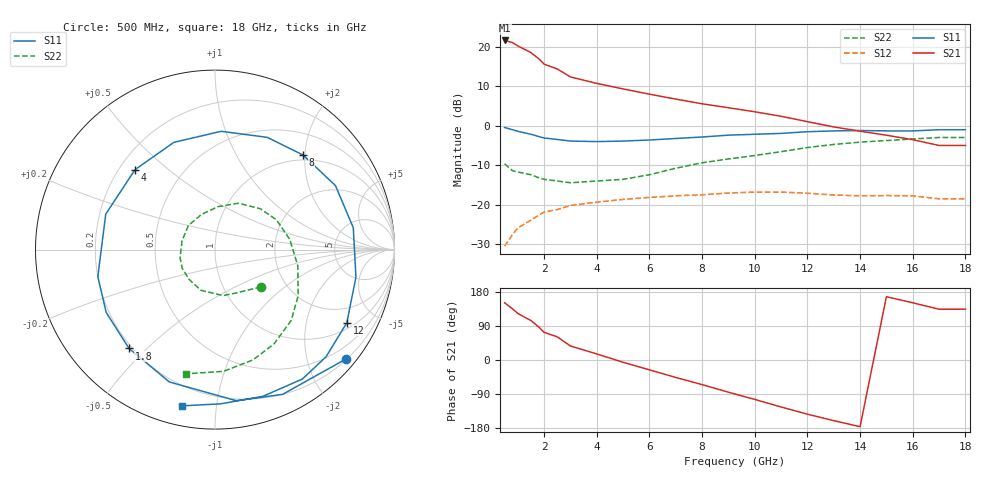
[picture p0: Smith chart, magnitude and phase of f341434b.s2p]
!ATF-34143
!S-PARAMETERS at Vds=4V  Id=40mA.  LAST UPDATED 01-29-99
# ghz s ma r 50
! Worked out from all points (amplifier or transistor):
!   23 points, 500 MHz to 18 GHz, reference 50 ohm
!   highest |S21| = 21.6 dB at 500 MHz (marker M1)
!   |S21| within 3 dB of that: start of sweep to 1.478 GHz
!   unconditionally stable (mu >= 1): 4.499 GHz to end of sweep
!   at 1.5 GHz: K = 0.42, MSG = 21.2 dB, |S12| = -23.9 dB
!   at 7 GHz: K = 1.12, MAG = 10.1 dB, |S12| = -17.7 dB
!   at 18 GHz: K = 1.33, MAG = 3.3 dB, |S12| = -18.5 dB
!   lowest NFmin = 0.10 dB at 500 MHz
!   S11 on the Smith chart (normalised r, x): 500 MHz: 0.22, -2.73; 1.8 GHz: 0.19, -0.44; 4 GHz: 0.26, +0.39; 8 GHz: 0.90, +1.96; 12 GHz: 1.25, -3.45; 18 GHz: 0.10, -0.81
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0.5  0.95 -40.0  11.97 151.0  0.03 68.0  0.33 -39.0
0.8  0.89 -65.0  11.25 135.0  0.042 56.0  0.27 -63.0
1  0.85 -82.0  10.22 123.0  0.051 48.0  0.26 -80.0
1.5  0.78 -109.0  8.405 104.0  0.064 36.0  0.24 -109.0
1.8  0.73 -131.0  7.024 87.0  0.074 27.0  0.22 -131.0
2  0.7 -150.0  6.002 73.0  0.081 19.0  0.21 -150.0
2.5  0.67 -167.0  5.223 61.0  0.087 12.0  0.2 -167.0
3  0.64 162.0  4.141 37.0  0.098 -1.0  0.19 165.0
4  0.63 135.0  3.428 16.0  0.108 -13.0  0.2 138.0
5  0.64 111.0  2.923 -6.0  0.117 -27.0  0.21 111.0
6  0.66 87.0  2.506 -26.0  0.124 -41.0  0.24 86.0
7  0.69 65.0  2.173 -46.0  0.13 -54.0  0.29 63.0
8  0.72 47.0  1.894 -65.0  0.134 -68.0  0.34 42.0
9  0.76 28.0  1.689 -85.0  0.141 -82.0  0.38 26.0
10  0.78 9.0  1.501 -104.0  0.145 -97.0  0.42 8.0
11  0.8 -11.0  1.317 -124.0  0.145 -113.0  0.47 -11.0
12  0.84 -29.0  1.125 -143.0  0.14 -128.0  0.53 -29.0
13  0.86 -44.0  0.966 -160.0  0.133 -141.0  0.58 -43.0
15  0.86 -72.0  0.759 167.0  0.131 -165.0  0.65 -71.0
16  0.86 -88.0  0.666 151.0  0.13 -180.0  0.68 -86.0
17  0.89 -102.0  0.563 134.0  0.119 168.0  0.71 -103.0
18  0.89 -102.0  0.563 134.0  0.119 168.0  0.71 -103.0
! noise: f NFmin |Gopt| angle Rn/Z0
0.5  0.1  0.87  13  0.16
0.9  0.13  0.82  27  0.14
1.5  0.17  0.73  49  0.11
1.8  0.2  0.7  60  0.1
2.5  0.28  0.6  85  0.07
3  0.34  0.54  104  0.05
5  0.57  0.4  180  0.03
6  0.69  0.38  -144  0.05
8  0.94  0.43  -82  0.2
10  1.19  0.62  -40  0.47
